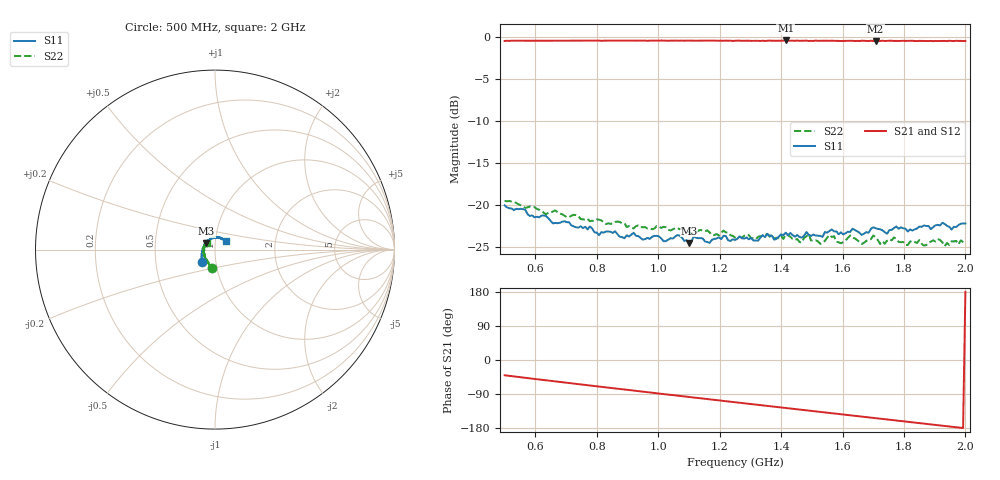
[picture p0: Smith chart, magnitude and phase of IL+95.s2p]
!Agilent Technologies,E8361C,US49010292,A.09.42.06
!Agilent E8361C: A.09.42.06
!Date: Friday, January 10, 2025 02:32:35
!Correction: S11(Full 2 Port(1,2))
!S21(Full 2 Port(1,2))
!S12(Full 2 Port(1,2))
!S22(Full 2 Port(1,2))
!S2P File: Measurements: S11, S21, S12, S22:
# Hz S  dB  R 50
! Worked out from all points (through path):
!   201 points, 500 MHz to 2 GHz, reference 50 ohm
!   highest |S21| = -0.39 dB at 1.415 GHz (marker M1); lowest = -0.5 dB at 1.708 GHz (marker M2)
!   group delay of S21, straight-line fit = 258 ps
!   lowest |S11| = -24.5 dB at 1.1 GHz (marker M3), VSWR 1.13, Z = 45.3 + j3.11 ohm
!   |S11| at or under -10 dB: start of sweep to end of sweep
!   |S22| runs from -24.9 to -19.5 dB; largest |S21 - S12| = 0.0065
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5e8  -20.03 -135.2  -0.44 -40.3  -0.43 -40.4  -19.50 -99.6
7.55e8  -22.74 -167.8  -0.41 -65.2  -0.42 -65.2  -21.70 -116.3
8.9e8  -23.96 174.0  -0.41 -77.9  -0.39 -78.0  -22.16 -126.9
1.0025e9  -23.74 157.7  -0.41 -88.4  -0.42 -88.4  -22.58 -133.6
1.1e9  -24.50 144.9  -0.41 -97.6  -0.41 -97.6  -23.26 -142.1
1.115e9  -23.75 143.1  -0.42 -99.0  -0.41 -98.9  -23.41 -141.6
1.1675e9  -24.50 134.7  -0.41 -103.8  -0.41 -103.7  -23.25 -149.4
1.2125e9  -23.66 128.8  -0.42 -108.1  -0.40 -107.9  -23.03 -148.8
1.25e9  -24.14 124.2  -0.43 -111.3  -0.41 -111.5  -23.86 -153.9
1.415e9  -23.28 104.5  -0.39 -126.7  -0.42 -126.7  -23.49 -166.8
1.4675e9  -23.87 98.9  -0.43 -131.4  -0.42 -131.3  -24.45 -172.5
1.49e9  -23.52 96.4  -0.45 -133.6  -0.43 -133.5  -23.42 -177.1
1.505e9  -23.51 91.5  -0.45 -134.8  -0.43 -134.8  -24.26 -176.1
1.5275e9  -23.66 89.7  -0.43 -136.9  -0.42 -136.9  -24.62 -178.0
1.5575e9  -23.07 86.0  -0.43 -139.8  -0.43 -139.7  -23.56 178.9
1.595e9  -23.25 79.3  -0.45 -143.2  -0.43 -143.1  -24.55 174.5
1.625e9  -23.19 79.4  -0.43 -146.0  -0.44 -146.0  -23.62 174.1
1.6625e9  -23.55 72.3  -0.42 -149.3  -0.45 -149.5  -24.64 168.8
1.7075e9  -22.74 71.2  -0.47 -153.4  -0.43 -153.5  -23.78 163.1
1.7225e9  -22.87 66.9  -0.46 -154.8  -0.41 -154.6  -24.64 161.6
1.7525e9  -22.98 65.0  -0.42 -157.3  -0.44 -157.6  -24.06 164.9
2e9  -22.19 37.0  -0.45 179.8  -0.45 179.9  -24.68 138.2
